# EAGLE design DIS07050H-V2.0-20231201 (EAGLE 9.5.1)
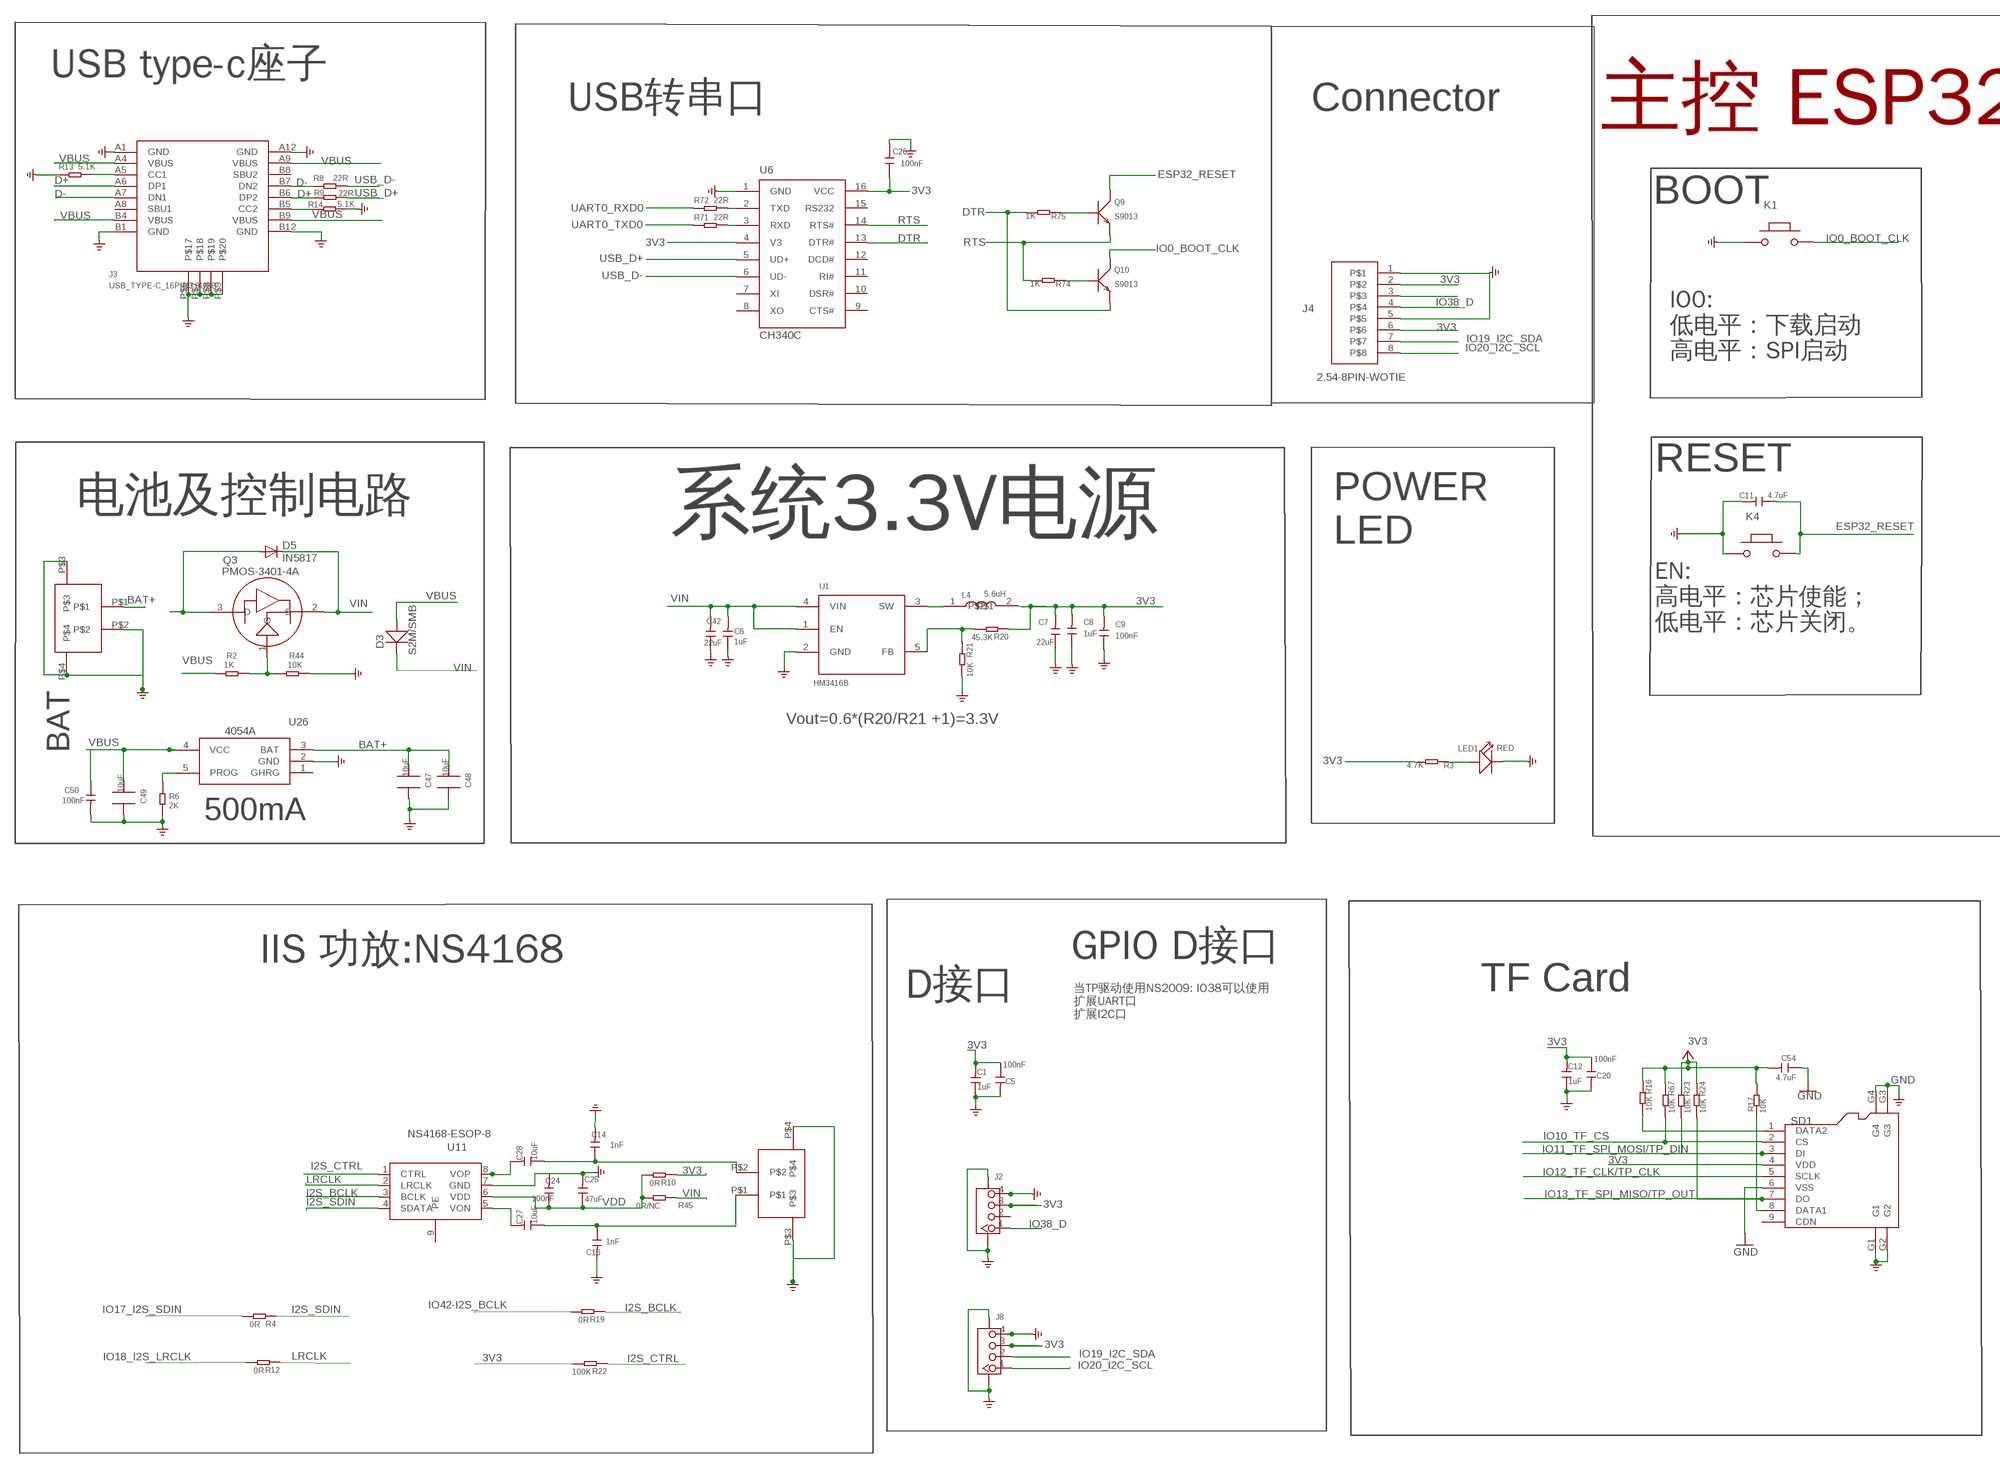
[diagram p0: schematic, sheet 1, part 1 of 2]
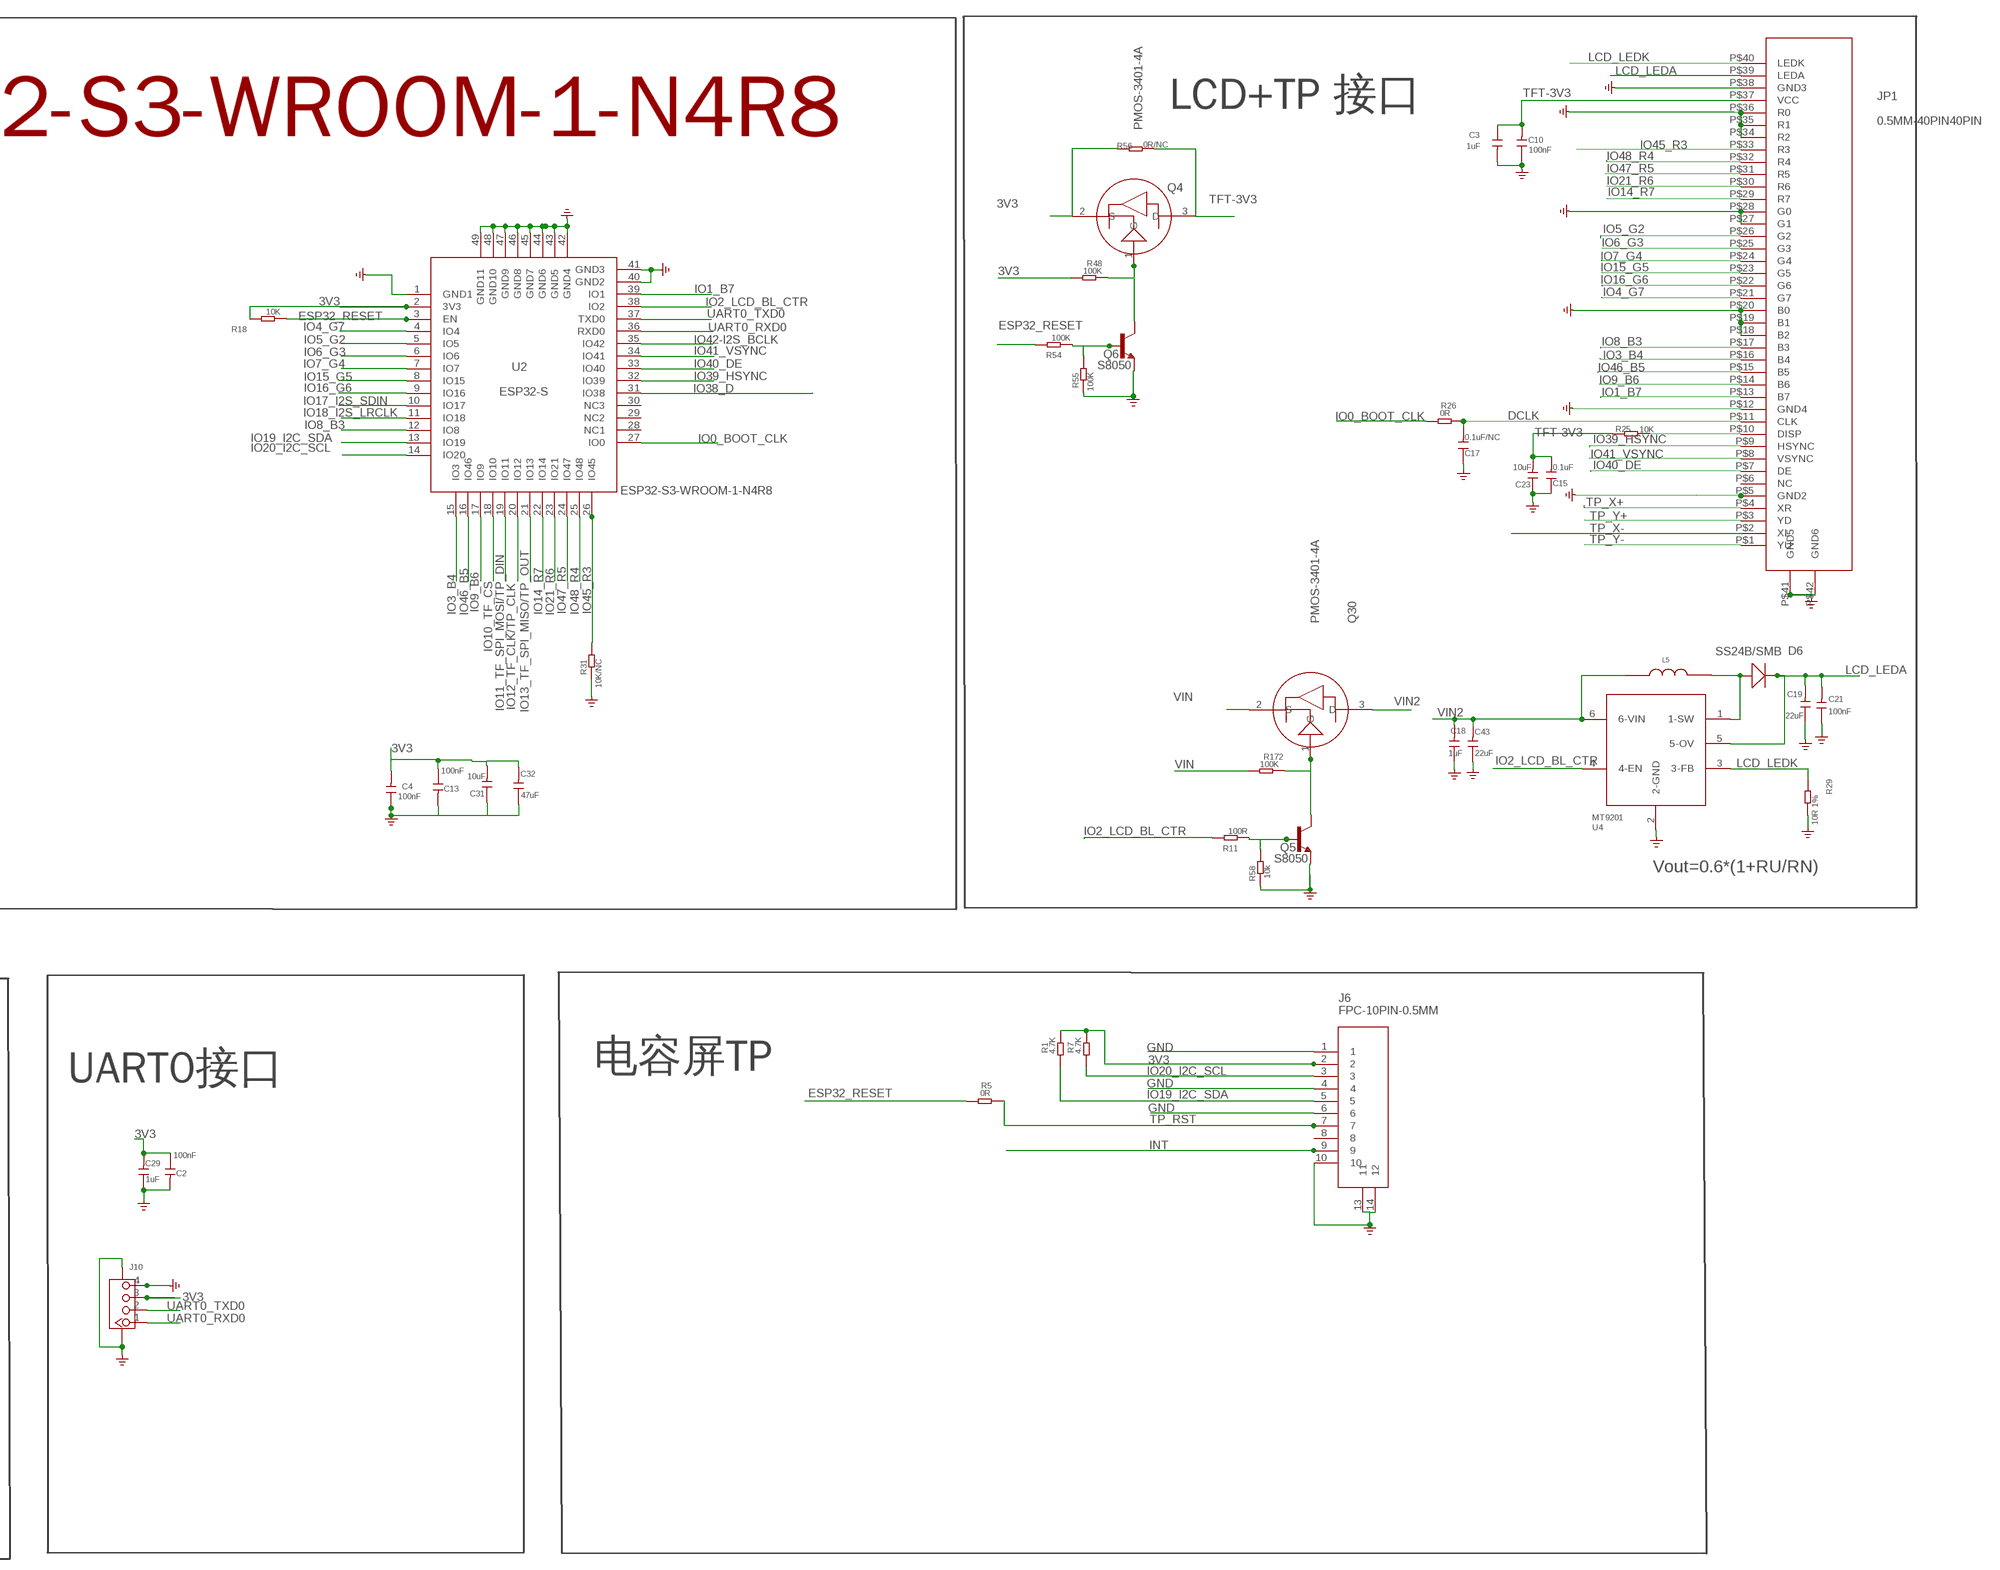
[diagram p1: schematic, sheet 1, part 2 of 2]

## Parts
C1  1uF  DISCRETE_C-0603  [DISCRETE_C0603]
C2  100nF  C-0603  [C0603]
C3  1uF  C-0603  [C0603]
C4  100nF  C-0603  [C0603]
C5  100nF  C-0603  [C0603]
C6  1uF  C0603  [0603]
C7  22uF  C0805  [0805]
C8  1uF  C0603  [0603]
C9  100nF  C0603  [0603]
C10  100nF  C-0603  [C0603]
C11  4.7uF  C0603  [0603]
C12  1uF  DISCRETE_C-0603  [DISCRETE_C0603]
C13  100nF  C-0603  [C0603]
C14  1nF  C-0603  [C0603]
C15  0.1uF  DISCRETE_C-0603  [DISCRETE_C0603]
C16  1nF  C-0603  [C0603]
C17  0.1uF/NC  DISCRETE_C-0603  [DISCRETE_C0603]
C18  1uF  C0603  [0603]
C19  22uF  C0805  [0805]
C20  100nF  C-0603  [C0603]
C21  100nF  C0603  [0603]
C23  10uF  DISCRETE_C-0603  [DISCRETE_C0603]
C24  100nF  C-0603  [C0603]
C25  47uF  C0805  [0805]
C26  100nF  C0603  [0603]
C27  10uF  DISCRETE_C-0603  [DISCRETE_C0603]
C28  10uF  DISCRETE_C-0603  [DISCRETE_C0603]
C29  1uF  DISCRETE_C-0603  [DISCRETE_C0603]
C31  10uF  DISCRETE_C-0603  [DISCRETE_C0603]
C32  47uF  C0805  [0805]
C42  22uF  C0805  [0805]
C43  22uF  C0805  [0805]
C47  10uF  C0805_S  [0805_S]
C48  10uF  C0805_S  [0805_S]
C49  10uF  C0805_S  [0805_S]
C50  100nF  C-0603  [C0603]
C54  4.7uF  DISCRETE_C-0603  [DISCRETE_C0603]
D3  S2M/SMB  214ABDO-214AB  [214AB]
D5  IN5817  DIODE-DO-214AC  [DO-214AC]
D6  SS24B/SMB  214ABDO-214AB  [214AB]
J1  PH2.0WT-2PIN  [PH2.0WT-2PIN]
J2  CONNECTOR_TWIG-4P-2.0-SMD-FEMALE-REINFORCE90D  [CONNECTOR_4P-SMD-2.0-90D]
J3  USB_TYPE-C_16PIN3.0USB  [KEVIN_3.0TYPEC-SMD]
J4  2.54-8PIN-WOTIE  [2.54-8P-WOTIE]
J5  PH2.0WT-2PIN  [PH2.0WT-2PIN]
J6  FPC-10PIN-0.5MM  [FPC-10PIN-0.5MM]
J8  CONNECTOR_TWIG-4P-2.0-SMD-FEMALE-REINFORCE90D  [CONNECTOR_4P-SMD-2.0-90D]
J10  CONNECTOR_TWIG-4P-2.0-SMD-FEMALE-REINFORCE90D  [CONNECTOR_4P-SMD-2.0-90D]
JP1  0.5MM-40PIN40PIN  [0.5MM*40P]
K1  BUTTON  PB157  [157SW]
K4  BUTTON  PB157  [157SW]
L4  5.6uH  L-0530  [CD54_CD54]
L5  CD32_6.8uH  CD32_950MA  [CD32]
LED1  RED  DISCRETE_LED0603  [DISCRETE_LED-0603]
Q3  PMOS-3401-4A  P-MOS-SOT23  [SOT-23]
Q4  PMOS-3401-4A  P-MOS-SOT23  [SOT-23]
Q5  S8050  SPARKFUN_TRANSISTOR_NPNSOT23  [SPARKFUN_SOT23]
Q6  S8050  SPARKFUN_TRANSISTOR_NPNSOT23  [SPARKFUN_SOT23]
Q9  S9013  TRANSISTOR-NPN-SOT23  [SOT23@1]
Q10  S9013  TRANSISTOR-NPN-SOT23  [SOT23@1]
Q30  PMOS-3401-4A  P-MOS-SOT23  [SOT-23]
R1  4.7K  R-0603  [R0603]
R2  1K  DISCRETE_R-0603  [DISCRETE_R0603]
R3  4.7K  DISCRETE_R-0603  [DISCRETE_R0603]
R4  0R  DISCRETE_R-0603  [DISCRETE_R0603]
R5  0R  R-0603  [R0603]
R6  2K  DISCRETE_R-0603  [DISCRETE_R0603]
R7  4.7K  R-0603  [R0603]
R8  22R  DISCRETE_R-0603  [DISCRETE_R0603]
R9  22R  DISCRETE_R-0603  [DISCRETE_R0603]
R10  0R  DISCRETE_R-0603  [DISCRETE_R0603]
R11  100R  R0603  [R0603]
R12  0R  DISCRETE_R-0603  [DISCRETE_R0603]
R13  5.1K  DISCRETE_R-0603  [DISCRETE_R0603]
R14  5.1K  DISCRETE_R-0603  [DISCRETE_R0603]
R16  10K  DISCRETE_R-0603  [DISCRETE_R0603]
R17  10K  DISCRETE_R-0603  [DISCRETE_R0603]
R18  10K  DISCRETE_R-0603  [DISCRETE_R0603]
R19  0R  DISCRETE_R-0603  [DISCRETE_R0603]
R20  45.3K  DISCRETE_R-0603  [DISCRETE_R0603]
R21  10K  DISCRETE_R-0603  [DISCRETE_R0603]
R22  100K  DISCRETE_R-0603  [DISCRETE_R0603]
R23  10K  DISCRETE_R-0603  [DISCRETE_R0603]
R24  10K  DISCRETE_R-0603  [DISCRETE_R0603]
R25  10K  DISCRETE_R-0603  [DISCRETE_R0603]
R26  0R  R-0603  [R0603]
R29  10R 1%  DISCRETE_R-0603  [DISCRETE_R0603]
R31  10K/NC  R0603  [R0603]
R44  10K  DISCRETE_R-0603  [DISCRETE_R0603]
R45  0R/NC  DISCRETE_R-0603  [DISCRETE_R0603]
R48  100K  R-0603  [R0603]
R54  100K  R0603  [R0603]
R55  100K  R0603  [R0603]
R56  0R/NC  DISCRETE_R-0603  [DISCRETE_R0603]
R58  10k  R0603  [R0603]
R67  10K  DISCRETE_R-0603  [DISCRETE_R0603]
R71  22R  DISCRETE_R-0603  [DISCRETE_R0603]
R72  22R  DISCRETE_R-0603  [DISCRETE_R0603]
R74  1K  DISCRETE_R-0603  [DISCRETE_R0603]
R75  1K  DISCRETE_R-0603  [DISCRETE_R0603]
R172  100K  R-0603  [R0603]
SD1  HOLDER-MICROSD-9P  [9P-SMD-W/-RING]
U1  HM3416B  A_XBJ_HM3420B  [A_XBJ_SOT23-5]
U2  ESP32-S  [ESP32-S3]
U4  MT9201  [SOT23-6]
U6  CH340C  CH340G  [SOP-16]
U11  NS4168-ESOP-8  [NS4168-ESOP-8]
U26  4054A  [SOP23-5]

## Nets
3V3: C1.2 C2.1 C4.2 C5.1 C7.2 C8.2 C9.2 C12.2 C13.1 C20.1 C26.1 C29.2 C31.2 C32.2 C54.2 J2.3 J4.2 J4.6 J6.2 J8.3 J10.3 L4.2 Q4.2(S) R1.2 R3.2 R7.2 R10.1 R16.1 R17.1 R18.1 R20.1 R22.2 R23.1 R24.1 R48.1 R56.1 R67.1 SD1.4(VDD) U2.2(3V3) U6.4(V3) U6.16(VCC) ; supply symbol labelled +3V3
BAT+: C47.2 C48.2 D5.A J1.P$1 Q3.3(D) U26.3(BAT)
D+: J3.A6(DP1) J3.B6(DP2) R9.1
D-: J3.A7(DN1) J3.B7(DN2) R8.1
DCLK: C17.2 JP1.P$11(CLK) R26.2
DTR: Q10.2(E) R75.2 U6.13(DTR#)
ESP32_RESET: C11.1 K4.2 Q9.3(C) R5.1 R18.2 R54.2 U2.3(EN)
GND: C1.1 C2.2 C3.2 C4.1 C5.2 C6.1 C7.1 C8.1 C9.1 C10.1 C11.2 C12.1 C13.2 C14.2 C15.1 C16.2 C17.1 C18.1 C19.1 C20.2 C21.1 C23.1 C24.2 C25.2 C26.2 C29.1 C31.1 C32.1 C42.1 C43.1 C47.1 C48.1 C49.1 C50.2 C54.1 J1.P$2 J1.P$3 J1.P$4 J2.4 J2.SS1 J2.SS2 J3.A1(GND) J3.A12(GND) J3.B1(GND) J3.B12(GND) J3.P$6 J3.P$7 J3.P$8 J3.P$9 J4.1 J4.5 J5.P$3 J5.P$4 J6.1 J6.4 J6.6 J6.10 J6.13 J6.14 J8.4 J8.SS1 J8.SS2 J10.4 J10.SS1 J10.SS2 JP1.P$5(GND2) JP1.P$12(GND4) JP1.P$18(B2) JP1.P$19(B1) JP1.P$20(B0) JP1.P$27(G1) JP1.P$28(G0) JP1.P$34(R2) JP1.P$35(R1) JP1.P$36(R0) JP1.P$38(GND3) JP1.P$41(GND5) JP1.P$42(GND6) K1.1 K4.1 LED1.- Q5.2(E) Q6.2(E) R6.2 R13.1 R14.2 R21.2 R29.2 R31.1 R44.1 R55.1 R58.1 SD1.6(VSS) SD1.G1 SD1.G2 SD1.G3 SD1.G4 U1.2(GND) U2.1(GND1) U2.40(GND2) U2.41(GND3) U2.42(GND4) U2.43(GND5) U2.44(GND6) U2.45(GND7) U2.46(GND8) U2.47(GND9) U2.48(GND10) U2.49(GND11) U4.2(2-GND) U6.1(GND) U11.7(GND) U26.2(GND)
I2S_BCLK: R19.1 U11.3(BCLK)
I2S_CTRL: R22.1 U11.1(CTRL)
I2S_SDIN: R4.1 U11.4(SDATA)
INT: J6.9
IO0_BOOT_CLK: K1.2 Q10.3(C) R26.1 U2.27(IO0)
IO1_B7: JP1.P$13(B7) U2.39(IO1)
IO2_LCD_BL_CTR: R11.2 U2.38(IO2) U4.4(4-EN)
IO3_B4: JP1.P$16(B4) U2.15(IO3)
IO4_G7: JP1.P$21(G7) U2.4(IO4)
IO5_G2: JP1.P$26(G2) U2.5(IO5)
IO6_G3: JP1.P$25(G3) U2.6(IO6)
IO7_G4: JP1.P$24(G4) U2.7(IO7)
IO8_B3: JP1.P$17(B3) U2.12(IO8)
IO9_B6: JP1.P$14(B6) U2.17(IO9)
IO10_TF_CS: R67.2 SD1.2(CS) U2.18(IO10)
IO11_TF_SPI_MOSI/TP_DIN: R23.2 SD1.3(DI) U2.19(IO11)
IO12_TF_CLK/TP_CLK: SD1.5(SCLK) U2.20(IO12)
IO13_TF_SPI_MISO/TP_OUT: R24.2 SD1.7(DO) U2.21(IO13)
IO14_R7: JP1.P$29(R7) U2.22(IO14)
IO15_G5: JP1.P$23(G5) U2.8(IO15)
IO16_G6: JP1.P$22(G6) U2.9(IO16)
IO17_I2S_SDIN: R4.2 U2.10(IO17)
IO18_I2S_LRCLK: R12.2 U2.11(IO18)
IO19_I2C_SDA: J4.7 J6.5 J8.2 R1.1 U2.13(IO19)
IO20_I2C_SCL: J4.8 J6.3 J8.1 R7.1 U2.14(IO20)
IO21_R6: JP1.P$30(R6) U2.23(IO21)
IO38_D: J2.1 J4.4 U2.31(IO38)
IO39_HSYNC: JP1.P$9(HSYNC) U2.32(IO39)
IO40_DE: JP1.P$7(DE) U2.33(IO40)
IO41_VSYNC: JP1.P$8(VSYNC) U2.34(IO41)
IO42-I2S_BCLK: R19.2 U2.35(IO42)
IO45_R3: JP1.P$33(R3) R31.2 U2.26(IO45)
IO46_B5: JP1.P$15(B5) U2.16(IO46)
IO47_R5: JP1.P$31(R5) U2.24(IO47)
IO48_R4: JP1.P$32(R4) U2.25(IO48)
LCD_LEDA: C19.2 C21.2 D6.2(-) JP1.P$39(LEDA) U4.5(5-OV)
LCD_LEDK: JP1.P$40(LEDK) R29.1 U4.3(3-FB)
LRCLK: R12.1 U11.2(LRCLK)
N$1: LED1.+ R3.1
N$2: C27.2 U11.5(VON)
N$3: C14.1 C28.1 J5.P$2
N$7: JP1.P$10(DISP) R25.2
N$8: C28.2 U11.8(VOP)
N$11: J3.A5(CC1) R13.2
N$13: L4.1 U1.3(SW)
N$15: C16.1 C27.1 J5.P$1
N$16: D6.1(+) L5.2 U4.1(1-SW)
N$17: J3.B5(CC2) R14.1
N$20: R20.2 R21.1 U1.5(FB)
N$21: Q3.1(G) R2.1 R44.2
N$22: R6.1 U26.5(PROG)
N$23: Q5.1(B) R11.1 R58.2
N$27: Q4.1(G) Q6.3(C) R48.2
N$28: J4.3
N$32: Q9.1(B) R75.1
N$33: Q6.1(B) R54.1 R55.2
N$36: Q5.3(C) Q30.1(G) R172.2
N$38: Q10.1(B) R74.1
N$40: R72.2 U6.2(TXD)
N$42: R71.2 U6.3(RXD)
N$47: R16.2 SD1.1(DATA2)
N$48: R17.2 SD1.8(DATA1)
RTS: Q9.2(E) R74.2 U6.14(RTS#)
TFT-3V3: C3.1 C10.2 C15.2 C23.2 JP1.P$37(VCC) Q4.3(D) R25.1 R56.2
TP_RST: J6.7 R5.2
TP_X+: JP1.P$4(XR)
TP_X-: JP1.P$2(XL)
TP_Y+: JP1.P$3(YD)
TP_Y-: JP1.P$1(YU)
UART0_RXD0: J10.1 R72.1 U2.36(RXD0)
UART0_TXD0: J10.2 R71.1 U2.37(TXD0)
USB_D+: R9.2 U6.5(UD+)
USB_D-: R8.2 U6.6(UD-)
VBUS: C49.2 C50.1 D3.1(+) J3.A4(VBUS) J3.A9(VBUS) J3.B4(VBUS) J3.B9(VBUS) R2.2 U26.4(VCC)
VDD: C24.1 C25.1 R10.2 R45.2 U11.6(VDD)
VIN: C6.2 C42.2 D3.2(-) D5.C Q3.2(S) Q30.2(S) R45.1 R172.1 U1.1(EN) U1.4(VIN)
VIN2: C18.2 C43.2 L5.1 Q30.3(D) U4.6(6-VIN)
Unconnected: J2.2 J3.A8(SBU1) J3.B8(SBU2) J6.8 JP1.P$6(NC) SD1.9(CDN) U2.28(NC1) U2.29(NC2) U2.30(NC3) U6.7(XI) U6.8(XO) U6.9(CTS#) U6.10(DSR#) U6.11(RI#) U6.12(DCD#) U6.15(RS232) U11.9(PE) U26.1(GHRG)

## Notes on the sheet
- USB type-c座子
- USB转串口 | Connector | LCD+TP 接口
- 主控 ESP32-S3-WROOM-1-N4R8
- BOOT
- IO0:
  低电平：下载启动
  高电平：SPI启动
- RESET
- 电池及控制电路
- 系统3.3V电源
- POWER
  LED
- EN:
  高电平：芯片使能；
  低电平：芯片关闭。
- Vout=0.6*(R20/R21 +1)=3.3V
- BAT
- Vout=0.6*(1+RU/RN)
- 500mA
- IIS 功放:NS4168 | GPIO D接口
- TF Card | UART0接口 | 电容屏TP
- D接口
- 当TP驱动使用NS2009: IO38可以使用
  扩展UART口
  扩展I2C口

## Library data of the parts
C1 C12 C27-C29 = A_xbj:DISCRETE_C*: Ceramic Capacitors
C2-C5 C10 C13 C14 C16 C20 C24 C50 = discrete:C*: Ceramic Capacitors
C6 C8 C9 C11 C18 C21 C26 = A_xbj:C0603
C7 C19 C25 C32 C42 C43 = A_xbj:C0805
C15 C17 C23 C31 C54 = A9G:DISCRETE_C*: Ceramic Capacitors
C47-C49 = CPT_SMD:C0805
D3 D6 = DO-214AB:214AB: 214AB
D5 = diode:DIODE-: DIODE
J1 J5 = cooper:PH2.0WT-2PIN
J2 J8 J10 = A_xbj:CONNECTOR_TWIG-4P-2.0-SMD-FEMALE-REINFORCE
J3 = WZ3532R024-ESP32-V0.1-20221226:USB_TYPE-C_16PIN
J4 = cooper:2.54-8PIN-WOTIE
J6 = cooper:FPC-10PIN-0.5MM
JP1 = cooper:0.5MM-40PIN
K1 K4 = MySMD:PB157
L4 = WZ2432R028-ESP32-V1.2-20231108:L-0530
L5 = CD54:CD32_950MA
LED1 = A_xbj:DISCRETE_LED*
Q3 Q4 Q30 = DFN8:P-MOS-SOT23
Q5 Q6 = Adafruit_HUZZAH32_ESP32_Feather:SPARKFUN_TRANSISTOR_NPN: Transistor NPN BJT configuration in SOT23 package. MMBT2222 is the common NPN we use. Double check BCE configuration again layout.
Q9 Q10 = discrete:TRANSISTOR-NPN*: NPN audion
R1 R5 R7 R26 R48 R172 = discrete:R*
R2 R6 R44 = A9G:DISCRETE_R*
R3 R4 R8-R10 R12-R14 R16-R25 R29 R45 R56 R67 R71 R72 R74 R75 = Crowtail-_LED-V2.0-20190615-01:DISCRETE_R*
R11 R31 R54 R55 R58 = cooper:R0603
SD1 = Connector:HOLDER-MICROSD-9P
U1 = CrowBot_-V1.0-20220525:A_XBJ_HM3420B
U2 = DW1000:ESP32-S; U2: ESP32-S3-WROOM-1-N4R8
U4 = cooper:MT9201
U6 = A_xbj:CH340G
U11 = STC_MCUSTC8G1K08A:NS4168-ESOP-8
U26 = DFN8:4054A

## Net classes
0 default: width 0.152 mm, drill 0.305 mm, clearance 0.203 mm

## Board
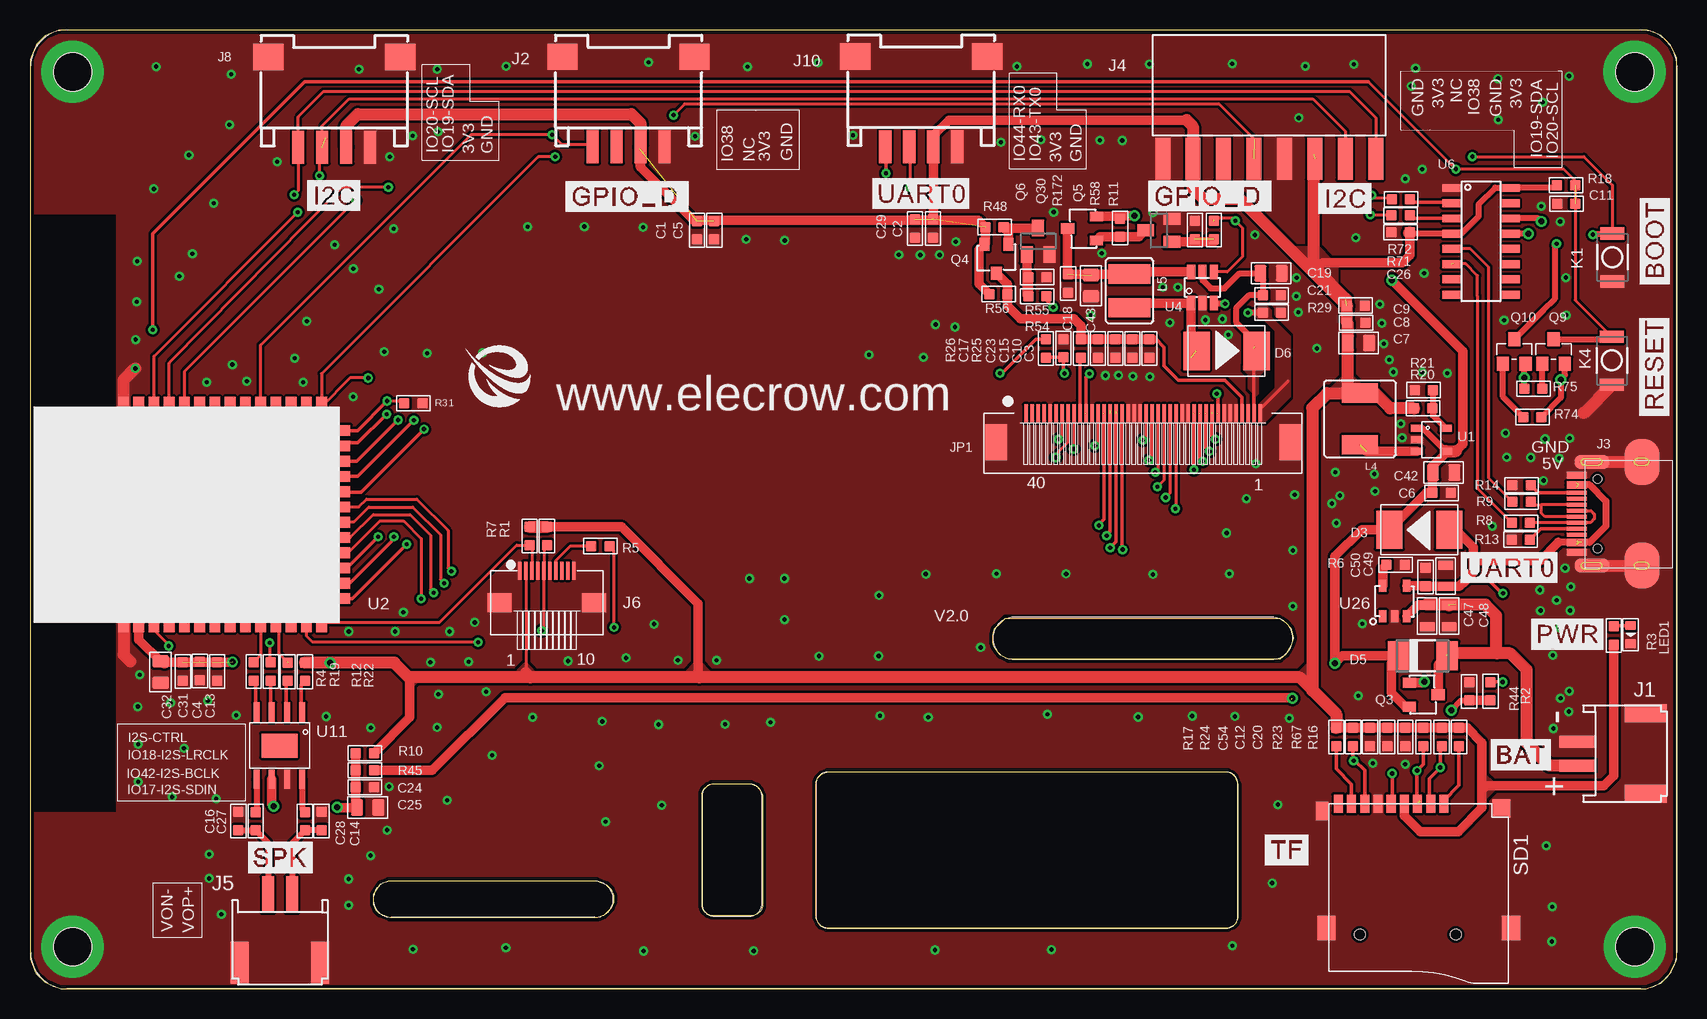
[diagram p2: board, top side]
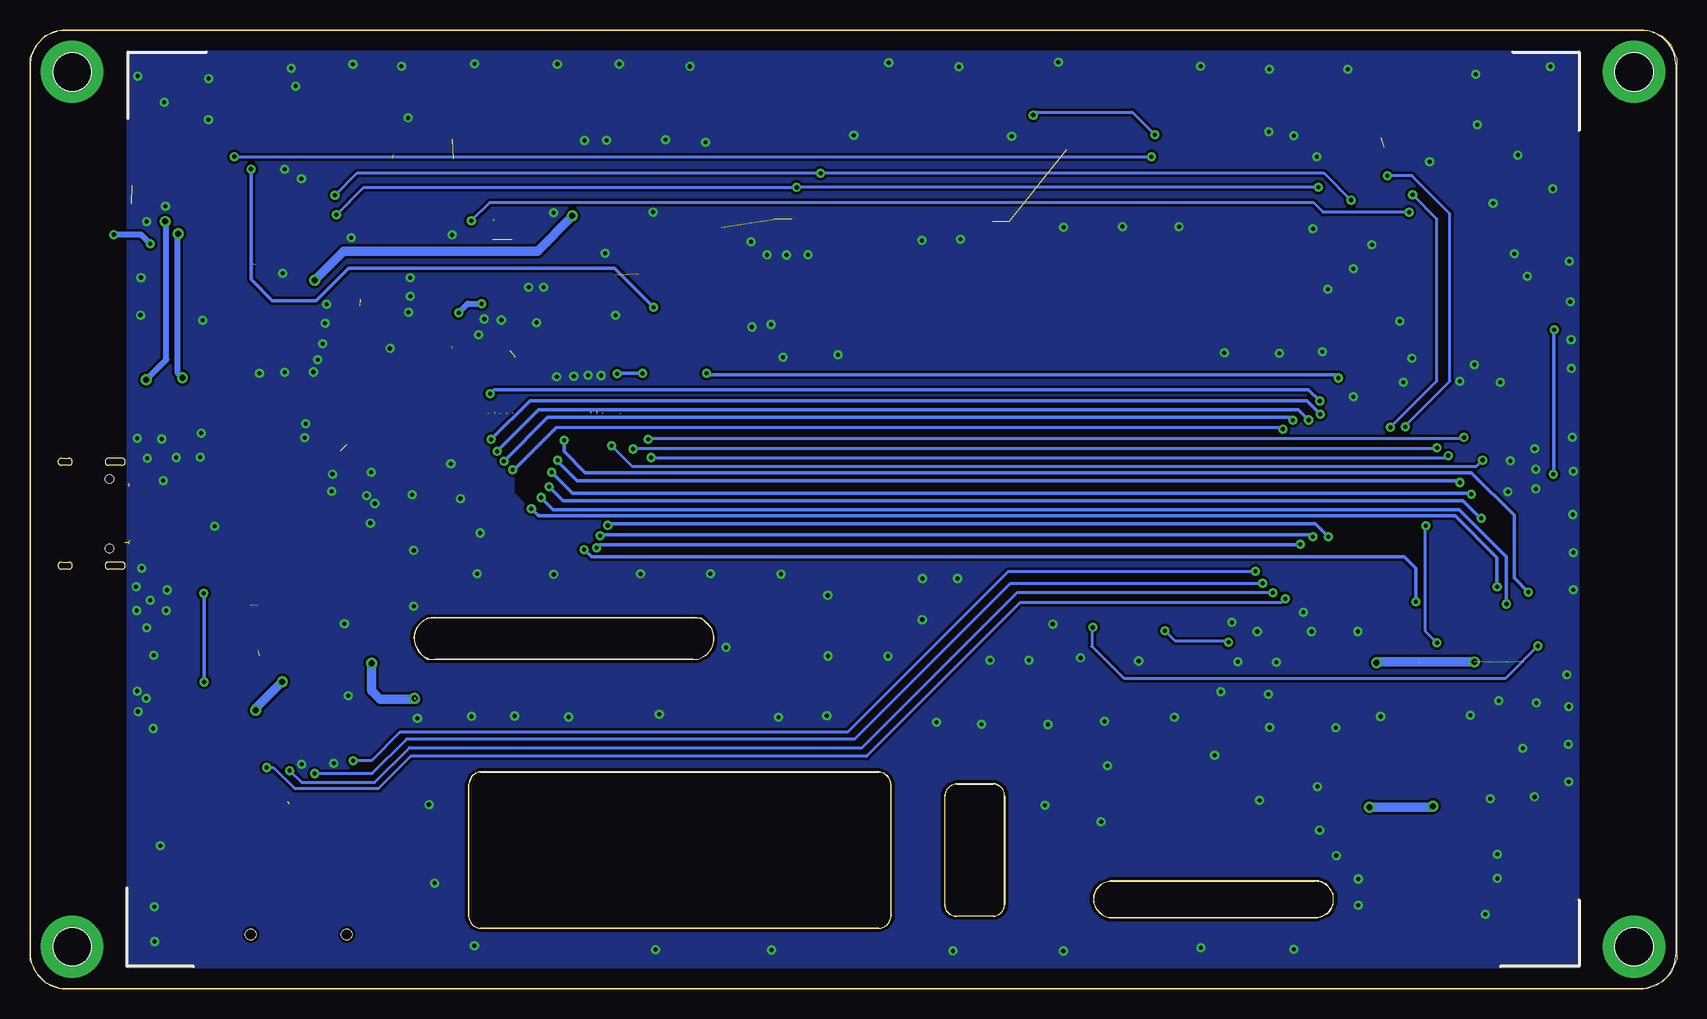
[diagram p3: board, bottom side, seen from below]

Size 137.27 x 79.91 mm. Coordinates in mm from the lower left corner, seen from the top.
Outline: 82 segments
Copper layers (1*16): Top 0.035mm / dielectric 1.5mm / Bottom 0.035mm
Design rules "default *": minimum track width 6mil, minimum drill 0.35mm, track to track 8mil, track to pad 7mil, pad to pad 7mil, via to via 8mil, smd to smd 10mil, copper to edge 10mil, drill to drill 8mil, minimum pad ring 10mil, minimum via ring 8mil, stop-mask expansion 4mil, vias tented up to drill 100mil, thermal gap 0mil

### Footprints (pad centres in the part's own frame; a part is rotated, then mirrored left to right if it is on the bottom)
DISCRETE_C0603 = smd 0.889 x 0.889: 1 -0.762,0; 2 0.762,0
C0603 = smd 0.889 x 0.889: 1 -0.762,0; 2 0.762,0
0603 = smd 0.889 x 0.889: 1 -0.762,0; 2 0.762,0
0805 = smd 1.016 x 1.397: 1 -0.889,0; 2 0.889,0
0805_S = smd 0.762 x 1.27: 1 -0.889,0; 2 0.889,0
214AB = smd 2.2 x 3.2: 1 -2.5,0; 2 2.5,0
DO-214AC = smd 1.8 x 2.4: A 2.025,0; C -2.025,0
PH2.0WT-2PIN = smd 1 x 3: P$1 -1,0; P$2 1,0 | smd 1.5 x 3.5: P$3 -3.35,-5.7; P$4 3.35,-5.7
CONNECTOR_4P-SMD-2.0-90D = smd 1.01 x 2.74: 1 -3,-0.1; 2 -1,-0.1; 3 1,-0.1; 4 3,-0.1 | smd 2.54 x 2.184: SS1 -5.5,7.4; SS2 5.5,7.4
KEVIN_3.0TYPEC-SMD = smd 0.3 x 1.7: A1 -3.35,0.5; A4 -2.55,0.5; A5 -1.25,0.5; A6 -0.25,0.5; A7 0.25,0.5; A8 1.25,0.5; A9 2.55,0.5; A12 3.35,0.5; B1 3.05,0.5; B4 2.25,0.5; B5 1.75,0.5; B6 0.75,0.5; B7 -0.75,0.5; B8 -1.75,0.5; B9 -2.25,0.5; B12 -3.05,0.5 | smd 1.143 x 2.921: P$6 -4.318,-0.762; P$7 4.318,-0.762 | smd 3.81 x 2.921: P$8 -4.318,-4.953; P$9 4.318,-4.953 | hole 0.68: -2.89,-1.22; 2.89,-1.22
2.54-8P-WOTIE = smd 1.25 x 3.5: 1 -8.839,-4.572; 2 -6.35,-4.572; 3 -3.81,-4.572; 4 -1.27,-4.572; 5 1.27,-4.572; 6 3.81,-4.572; 7 6.35,-4.572; 8 8.89,-4.572
FPC-10PIN-0.5MM = smd 0.3 x 1.5: 1 -2.25,2.54; 2 -1.75,2.54; 3 -1.25,2.54; 4 -0.75,2.54; 5 -0.25,2.54; 6 0.25,2.54; 7 0.75,2.54; 8 1.25,2.54; 9 1.75,2.54; 10 2.25,2.54 | smd 2 x 1.6: 13 -3.95,-0.14; 14 3.95,-0.14
0.5MM*40P = smd 0.3 x 1.5: P$1 -8.81,1.73; P$2 -8.31,1.73; P$3 -7.81,1.73; P$4 -7.31,1.73; P$5 -6.81,1.73; P$6 -6.31,1.73; P$7 -5.81,1.73; P$8 -5.31,1.73; P$9 -4.81,1.73; P$10 -4.31,1.73; P$11 -3.81,1.73; P$12 -3.31,1.73; P$13 -2.81,1.73; P$14 -2.31,1.73; P$15 -1.81,1.73; P$16 -1.31,1.73; P$17 -0.81,1.73; P$18 -0.31,1.73; P$19 0.19,1.73; P$20 0.69,1.73; P$21 1.19,1.73; P$22 1.69,1.73; P$23 2.19,1.73; P$24 2.69,1.73; P$25 3.19,1.73; P$26 3.69,1.73; P$27 4.19,1.73; P$28 4.69,1.73; P$29 5.19,1.73; P$30 5.69,1.73; P$31 6.19,1.73; P$32 6.69,1.73; P$33 7.19,1.73; P$34 7.69,1.73; P$35 8.19,1.73; P$36 8.69,1.73; P$37 9.19,1.73; P$38 9.69,1.73; P$39 10.19,1.73; P$40 10.69,1.73 | smd 1.8 x 3: P$41 -11.31,-0.67; P$42 13.19,-0.67
157SW = smd 1.016 x 1.981: 1 0,0; 2 4,0
CD54_CD54 = smd 3 x 1.6: 1 0,2.159; 2 0,-2.159
CD32 = smd 3.5 x 1.6: 1 0,1.409; 2 0,-1.409
DISCRETE_LED-0603 = smd 0.762 x 0.889: + -0.762,0; - 0.762,0
SOT-23 = smd 1.1 x 0.8: 1 1.2,-1; 2 1.2,1 | smd 1.1 x 0.9: 3 -1.2,0
SPARKFUN_SOT23 = smd 1 x 1.4: 1 -0.95,-1.1; 2 0.95,-1.1; 3 0,1.1
SOT23@1 = smd 1.016 x 1.143: 1 -0.95,-1.016; 2 0.95,-1.016; 3 0,1.016
R0603 = smd 0.889 x 0.889: 1 -0.762,0; 2 0.762,0
DISCRETE_R0603 = smd 0.889 x 0.889: 1 -0.762,0; 2 0.762,0
9P-SMD-W/-RING = smd 1.524 x 0.762: 1 0,4.4; 2 0,3.3; 3 0,2.2; 4 0,1.1; 5 0,0; 6 0,-1.1; 7 0,-2.2; 8 0,-3.3; 9 0,-4.4 | smd 1.524 x 1.016: G1 0.6,-5.746 | smd 2.032 x 1.524: G2 10.373,-5.4; G3 10.373,10 | smd 1.524 x 1.524: G4 0.392,9.181 | hole 0.889: 10.9,-2.6; 10.9,5.4
A_XBJ_SOT23-5 = smd 0.6 x 1: 1 -0.95,-1.2; 2 0,-1.2; 3 0.95,-1.2; 4 0.95,1.2; 5 -0.95,1.2
ESP32-S3 = smd 1.6 x 0.9: 1 0,18.01; 2 0,16.74; 3 0,15.47; 4 0,14.2; 5 0,12.93; 6 0,11.66; 7 0,10.39; 8 0,9.12; 9 0,7.85; 10 0,6.58; 11 0,5.31; 12 0,4.04; 13 0,2.77; 14 0,1.5; 27 18,1.5; 28 18,2.77; 29 18,4.04; 30 18,5.31; 31 18,6.58; 32 18,7.85; 33 18,9.12; 34 18,10.39; 35 18,11.66; 36 18,12.93; 37 18,14.2; 38 18,15.47; 39 18,16.74; 40 18,18.01 | smd 0.9 x 1.8: 15 2,0; 16 3.28,0; 17 4.55,0; 18 5.82,0; 19 7.09,0; 20 8.36,0; 21 9.63,0; 22 10.9,0; 23 12.17,0; 24 13.44,0; 25 14.71,0; 26 16,0 | smd 1 x 1: 41 7.64,11.16; 42 9.14,11.16; 43 6.14,11.16; 44 6.14,14.16; 45 7.64,12.66; 46 9.14,12.66; 47 7.64,14.16; 48 9.14,14.16; 49 6.14,12.66
SOT23-6 = smd 0.69 x 1.2: 1 -0.95,-1.3; 2 0,-1.3; 3 0.95,-1.3; 4 0.95,1.3; 5 0,1.3; 6 -0.95,1.3
SOP-16 = smd 0.66 x 1.5: 1 -4.445,-2.475; 2 -3.175,-2.475; 3 -1.905,-2.475; 4 -0.635,-2.475; 5 0.635,-2.475; 6 1.905,-2.475; 7 3.175,-2.475; 8 4.445,-2.475; 9 4.445,2.475; 10 3.175,2.475; 11 1.905,2.475; 12 0.635,2.475; 13 -0.635,2.475; 14 -1.905,2.475; 15 -3.175,2.475; 16 -4.445,2.475
NS4168-ESOP-8 = smd 1.6 x 0.5: 1 -2.8,1.905; 2 -2.8,0.635; 3 -2.8,-0.635; 4 -2.8,-1.905; 5 2.8,-1.905; 6 2.8,-0.635; 7 2.8,0.635; 8 2.8,1.905 | smd 2 x 3: 9 0,0
SOP23-5 = smd 1 x 0.635: 1 -1.27,1; 2 -1.27,0; 3 -1.27,-1; 4 1.27,-1; 5 1.27,1

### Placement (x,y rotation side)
C1  55.61,63.22 90 top
C2  75.26,63.36 270 top
C3  93.32,53.37 270 top
C4  14.17,26.48 90 top
C5  57.04,63.22 270 top
C6  117.67,41.33 180 top
C7  110.74,53.82 180 top
C8  110.54,55.51 180 top
C9  110.52,56.94 180 top
C10  91.9,53.37 90 top
C11  128.07,65.42 180 top
C12  113.15,20.99 90 top
C13  15.61,26.44 270 top
C14  24.29,13.99 90 top
C15  90.47,53.37 90 top
C16  17.37,13.99 90 top
C17  86.15,53.4 270 top
C18  86.54,58.78 90 top
C19  103.45,59.63 180 top
C20  114.65,20.99 270 top
C21  103.52,57.79 180 top
C23  89.03,53.37 90 top
C24  27.91,16.8 0 top
C25  28.15,15.11 0 top
C26  114.26,63.05 180 top
C27  18.81,13.97 90 top
C28  22.92,13.97 90 top
C29  73.76,63.36 90 top
C31  12.74,26.45 90 top
C32  10.89,26.4 90 top
C42  117.84,43.03 180 top
C43  88.44,58.6 90 top
C47  116.46,31.08 90 top
C48  118.29,31.07 90 top
C49  118.01,34.42 270 top
C50  116.33,34.32 90 top
C54  111.71,20.99 90 top
D3  115.81,38.26 180 top
D5  116.1,27.75 0 top
D6  99.74,53.16 0 top
J1  128.97,19.61 90 top
J2  49.9,70.28 0 top
J3  129.44,39.6 90 top
J4  103.29,73.77 0 top
J5  20.83,7.88 0 top
J6  43.08,32.31 0 top
J8  25.36,70.25 0 top
J10  74.29,70.29 0 top
JP1  91.84,46.23 0 top
K1  131.9,58.95 90 top
K4  131.86,50.34 90 top
L4  110.87,47.5 180 top
L5  91.67,58.17 0 top
LED1  133.43,29.52 270 top
Q3  116.18,24.51 180 top
Q4  80.56,60.85 90 top
Q5  94.1,63.22 90 top
Q6  84.04,62.3 0 top
Q9  127,53.12 0 top
Q10  123.72,53.12 0 top
Q30  87.7,63.37 0 top
R1  43.08,37.74 90 top
R2  121.74,24.8 90 top
R3  132.03,29.46 270 top
R4  18.66,26.45 90 top
R5  47.54,36.9 180 top
R6  113.84,35.36 0 top
R7  41.66,37.74 90 top
R8  124.27,38.85 180 top
R9  124.32,40.59 180 top
R10  27.91,19.64 180 top
R11  98.69,63.24 90 top
R12  21.47,26.43 90 top
R13  124.27,37.45 0 top
R14  124.33,41.98 180 top
R16  119.12,20.99 270 top
R17  108.89,20.99 270 top
R18  128.05,66.96 0 top
R19  20.08,26.45 90 top
R20  116.12,48.38 0 top
R21  116.18,49.9 180 top
R22  22.92,26.43 90 top
R23  116.15,20.99 270 top
R24  110.28,20.99 270 top
R25  87.6,53.37 270 top
R26  84.68,53.37 270 top
R29  103.52,56.36 0 top
R31  31.97,48.8 180 top
R44  119.96,24.8 270 top
R45  27.91,18.22 180 top
R48  80.4,63.48 0 top
R54  83.97,57.72 0 top
R55  83.98,59.32 180 top
R56  80.73,57.91 0 top
R58  97.09,63.24 270 top
R67  117.68,20.99 270 top
R71  114.25,64.45 0 top
R72  114.28,65.8 0 top
R74  125.24,47.66 0 top
R75  125.32,50.01 180 top
R172  90.87,63.42 270 top
SD1  113.46,15.44 270 top
U1  116.81,45.76 270 top
U2  25.81,30.53 90 top
U4  97.74,58.45 0 top
U6  120.95,62.3 270 top
U11  20.8,20.27 270 top
U26  113.76,32.32 90 top
U$30  [ELECROW-NEW]  36.28,48.48 0 top
U$33  [5.0底框]  138.34,-0.06 0 bottom
U$41  [5.0板框]  -0.6,0.03 0 top

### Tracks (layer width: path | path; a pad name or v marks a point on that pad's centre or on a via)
0
  cutout Bottom: 93.15,46.48 96.51,46.48 96.76,46.23 96.76,41.36 95.08,39.68 95.08,41.78 93.06,43.79 93.06,46.4
3V3  (via drill 0.5)  (9 unrouted)
  Top 0.203: 109.65,56.95 C9.2 109.53,56.83 | C8.2 109.55,55.54
  Top 0.254: J6.2 41.33,26.31 41.33,25.97 41.4,25.9
  Top 0.5: U6.16 123.45,66.77 | C26.1 115.13,62.93 U6.4 119.32,62.93 120.75,64.36 120.75,65.37 122.15,66.77 123.45,66.77 | R18.1 127.09,66.77 123.45,66.77
  Top 0.8: C32.2 9.07,29.12 U2.2 | SD1.4 114.56,14.45 115.9,13.11 119.04,13.11 121.04,15.1 121.04,16.58 | 50.85,69.96 50.85,68.53 50.9,68.48 | J10.3 75.32,70.23 | 75.32,70.23 75.32,64.18 C2.1 | 96.42,72.4 76.6,72.4 75.32,71.12 75.32,70.23 | 50.9,68.48 55.32,64.06 79.06,64.06 R48.1 79.64,62.13 Q4.2 79.1,61.59 79.1,58.77 R56.1 | 50.9,68.48 J2.3 | R17.1 R24.1 C54.2 C12.2 C20.1 R23.1 R67.1 R16.1 119.81,21.75 121.04,20.52 121.04,16.58 | R1.2 43.67,38.51 43.68,38.5 49.3,38.5 55.68,32.12 55.68,26.07 55.8,25.95 55.85,25.9 | v16.88,27.24 16.84,27.21 11.23,27.21 | 31.66,25.9 31.66,22.63 R10.1 | 121.04,16.58 121.4,16.94 131.19,16.94 132.03,17.78 R3.2 | 107.22,59.96 107.77,60.51 114.4,60.51 115.02,61.13 C26.1
  Top 1: 11.23,27.21 11.14,27.29 C32.2 | 114.97,63 C26.1 | R22.2 v25.02,27.19 30.37,27.19 31.66,25.9 31.71,25.95 41.7,25.95 | R7.2 R1.2 | 109.71,57.47 107.22,59.96 107.01,60.17 107.01,69.52 | 110.37,49.66 109.85,50.18 C7.2 109.85,55.44 C8.2 109.78,56.92 C9.2 100.91,65.79 97.87,65.79 96.94,66.72 J4.2 96.94,71.88 96.42,72.4 | J8.3 26.36,71.93 27.33,72.9 50.14,72.9 50.9,72.14 J2.3 | 41.7,25.95 55.8,25.95 105.85,25.95 108.89,22.91 R17.1 108.89,22.87 106.88,24.87 106.88,48.41 108.13,49.66 110.37,49.66 | 41.7,25.95 41.33,26.31 | 110.37,49.66 L4.2 | R20.1 113.39,48.38 112.07,49.71 110.42,49.71 110.37,49.66
  Bottom 0.8: v25.02,27.19 24.97,27.24 v16.88,27.24 | v16.88,27.24
  pour Top (no thermals): 107.09,60.26 109.02,60.26 109.02,58.24 107.09,60.17
  pour Top (no thermals): 106.67,27.33 105.41,26.07 106.84,24.64 106.84,27.41 106.76,27.41
  pour Top (no thermals): 31.49,24.72 32.42,25.65 31.49,26.57
  pour Top (no thermals): 121.12,15.57 122.38,16.83 120.95,18.26 120.95,15.48 121.04,15.48
  pour Top (no thermals): 56.94,26.24 55.68,27.5 54.26,26.07 57.03,26.07 57.03,26.15
  pour Top (no thermals): 42.58,25.98 41.32,27.24 39.89,25.82 42.66,25.82 42.66,25.9
  pour Top (no thermals): 111.12,50.26 109.86,51.52 108.44,50.09 111.21,50.09 111.21,50.18
  pour Top (no thermals): 105.09,61.91 107.02,61.91 107.02,59.89 105.09,61.82
  pour Top (no thermals): 108.91,60.32 106.98,60.32 106.98,62.33 108.91,60.4
BAT+  (2 unrouted)
  Top 0.8: C48.2 118.3,31.96 | C47.2 115.68,31.97 U26.3 115.72,32.01 116.43,32.01 | 118.87,32.01 118.29,32.01 | Q3.3 117.38,27.01 D5.A
  Top 1: J1.P$1 126.65,18.61 124.75,20.5 124.75,26.6 123.39,27.97 122.3,27.97 | 122.3,27.97 118.26,27.97 118.26,28.17 | 122.3,27.97 122.23,28.04 122.23,31.11 121.33,32.01 118.29,32.01 | C48.2 118.24,32.01 116.43,32.01
D+
  Top 0.254: J3.A6 126.29,39.35 125.98,39.65 125.98,40.3 | J3.B6 125.98,40.34 125.98,40.3 | 125.98,40.3 125.37,40.3 R9.1
D-
  Top 0.254: R8.1 J3.B7 130.09,38.85 130.4,39.17 130.4,39.57 130.13,39.85 J3.A7
DCLK  (via drill 0.35)  (1 unrouted)
  Top 0.3: R26.2 84.71,52.63 C17.2 86.16,51.35 v86.22,51.29 | v88.32,51.26 88.03,50.97 88.03,47.91
  Bottom 0.3: v88.32,51.26 88.3,51.29 v86.22,51.29
DTR  (via drill 0.5)
  Top 0.5: R75.2 v124.56,50.93 124.56,51.98 Q10.2 | v124.9,62.94 124.89,62.93 U6.13
  Bottom 0.5: v124.9,62.94 124.98,62.87 124.98,51.35 v124.56,50.93
ESP32_RESET  (via drill 0.35)  (1 unrouted)
  Top 0.152: 131.84,54.36 K4.2
  Top 0.254: K4.2 128.81,57.39 R18.2 128.81,67.35 127.84,68.32 v118.85,68.32 111.56,75.61 | U2.3 10.34,29.9 11.57,28.66 v11.57,28.58 | R5.1 48.63,36.57 48.63,30.17 v48.68,30.12
  Top 0.3: v10.28,42.89 10.28,30.59 U2.3 | 111.56,75.61 22.88,75.61 10.22,62.95 v10.22,54.92 | v85.29,56.81 84.74,57.37 R54.2
  Top 0.5: Q9.3 131.65,54.13 K4.2
  Bottom 0.254: v48.68,30.12 48.76,30.2 48.76,28.55 46.1,25.89 14.26,25.89 v11.57,28.58
  Bottom 0.3: v10.28,42.89 10.26,42.91 10.26,54.88 v10.22,54.92 | v118.85,68.32 118.85,59.13 117.07,57.35 113.41,57.35 110.72,60.05 88.53,60.05 v85.29,56.81
GND  (via drill 0.35, 3.2 pad 5.2)
  Top 1: v8.78,51.7 7.8,50.72 U2.40 7.8,45.62 8.1,45.31 | 7.9,33.3 7.8,33.2 U2.1 7.8,27.87 8.38,27.28 | J3.P$7 J3.P$9 | J3.P$6 J3.P$8 | K4.1 129.51,47.99
  other vias: 133.76,76.43 3.56,76.43 3.56,3.51 133.77,3.51 91.94,51.05 75.83,61.17 127.55,63.94 105.27,36.54 52.66,15.32 115.13,75.23 22.78,50.56 69.93,52.84 100.23,3.6 102.09,62.83 82.26,76.87 13.54,61.26 95.03,55.53 84.81,22.88 55.44,71.06 126.16,42.36 29.99,69.34 11.86,16 106.31,76.89 46.21,63.53 41.89,22.63 65.76,27.74 99.75,37.99 15.96,6.21 9.02,17.25 105.28,31.9 26.95,49.35 26.55,9.16 89.19,70.73 126.29,45.83 105.56,57.73 85.13,3.28 100.22,77.11 113.64,51.41 89.66,51.11 14.83,24.02 127.49,44.22 74.87,22.63 91.05,70.7 88.14,77.08 114.28,47.1 111.06,30.42 92.38,22.66 27.42,76.63 115.5,76.73 93.36,51.02 74.49,52.64 34.01,71.43 30.32,63.34 75.45,3.24 93.31,77.07 33.11,52.96 108.52,40.45 47.7,22.29 33.95,76.64 88.45,56.13 123.09,44.3 77.17,62.27 29.08,58.31 57.95,22.06 110.73,24.44 122.39,72.44 93.61,34.54 65.69,77.18 100.45,22.71 13.86,44 39.69,76.88 33.38,27.23 72.42,61.19 112.12,41.46 105.72,56.39 8.99,23.53 90.75,51.14 102.19,43.77 29.54,53.1 126.99,21.7 8.81,54.11 52.01,30.41 52.41,22.04 74.21,61.16 128.38,31.53 116.05,68.32 128.34,45.89 15.31,65.47 24.68,22.7 47.45,18.59 101.39,40.86 38.52,19.47 99.99,34.61 70.75,27.74 34.05,24.55 70.85,22.76 13.25,69.49 11.72,23.83 26.56,6.98 17.2,22.79 125.98,65.22 33.93,21.79 20.61,68.93 41.48,63.52 38.01,24.77 59.82,76.85 28.41,21.77 80.56,34.59 79.25,28.46 59.7,62.46 112.05,42.9 114.38,45.92 8.63,33.26 8.63,36.36 8.68,39.53 8.63,43.14 8.7,45.96 95.69,58.46 97.97,55.74 99.4,55.82 77.09,55.16 75.5,55.37 51.55,77.23 109.2,41.11 99.88,54.5 94.45,58.46 14.07,41.42 47.98,13.92 11.75,43.32 49.69,27.58 11.74,41.66 9.03,20.4 12.84,20.06 8.89,57.27 128.26,23.11 8.95,60.64 128.32,24.82 12.46,59.38 59.97,34.2 9.15,26.17 108.82,43.06 31.12,31.4 112.87,53.77 15.53,15.84 54,27.39 62.91,62.37 108.89,38.82 14.95,11.22 126.95,27.8 14.94,9.21 104.01,15.36 39.66,3.43 51.14,3.16 31.92,3.32 70.77,32.79 111.94,18.81 74.67,34.57 85.33,64.74 61.72,22.22 16.63,72 62.9,30.78 80.95,70.56 31.9,71.11 107.26,53.37 114.64,67.51 93.62,64.68 105.58,59.27 84.28,70.75 125.09,44.28 16.77,76.23 126.09,73.88 122.99,46.32 128.02,59.28 128.05,56.15 122.88,55.72 37.72,53.02 68.6,71.14 36.57,27.27 60.33,3.17 51.11,63.48 86.37,34.58 28.39,11.11 44.85,27.32 62.88,34.2 121.88,38.55 126.86,3.95 127.58,24.23 103.55,8.82 122.37,75.86 110.35,77.06 116.21,59.65 112.53,57.04 112.68,55.47 10.53,76.86 10.33,66.66 127.53,30.09 105.42,41.18 128.43,33.52 125.85,33.24 127.25,32.39 125.91,31.53 127.96,35.07 126.4,11.92 126.9,6.85 26.96,60.02 22.07,52.56 23.08,55.63 89.34,61.3 128.3,76.07 34.77,15.73 37.08,30.54 30.44,29.79 34.98,29.79 26.58,29.79 29.77,13.24 29.95,16.86 11.85,45.01 114.63,18.73 104.98,22.56 96.88,22.74 118.15,51.3 113.3,52.43 116.05,51.39 14.72,50.56 18.08,50.64 16.87,52.03 25.4,62.01 110.51,62.6 105.76,72.58 57.23,27.38
  pour Bottom: 8.19,78.05 129.11,78.05 129.11,1.84 8.19,1.84
  pour Top (rank 4): -0.01,79.91 137.25,79.91 137.25,-0.06 -0.09,-0.06 -0.09,14.73 7.22,14.73 7.22,64.54 -0.01,64.54
I2S_BCLK
  Top 0.3: U11.3 20.08,23.15 R19.1
I2S_CTRL
  Top 0.3: U11.1 22.62,23.15 22.62,25.36 R22.1
I2S_SDIN
  Top 0.3: U11.4 18.81,23.15 18.81,25.54 R4.1
IO0_BOOT_CLK  (via drill 0.35)
  Top 0.254: v43.79,69.33 42.36,69.33 24.31,51.28 U2.27 26.69,50.91 v28.2,50.91 | v120.23,69.36 129.53,69.36 131.9,66.99 K1.2
  Top 0.3: v80.87,51.3 81.03,51.3 83.87,54.13 R26.1
  Top 0.5: Q10.3 126.16,56.57 127.08,57.49 127.08,61.94 v127.25,62.1 | v130.28,62.86 130.36,62.94 132.29,62.94 132.28,62.95 K1.2
  Bottom 0.254: v120.23,69.36 v120.23,69.35 43.81,69.35 v43.79,69.33
  Bottom 0.3: v80.87,51.3 80.73,51.16 28.45,51.16 v28.2,50.91
  Bottom 0.5: v127.25,62.1 128.01,62.86 v130.28,62.86
IO1_B7  (via drill 0.35)
  Top 0.254: JP1.P$13 89.03,45.34 88.94,45.25 v88.79,45.25 | U2.39 9.07,47.14 10.16,46.05 14.2,46.05 v16.19,44.07
  Bottom 0.254: v88.79,45.25 87.1,43.56 16.69,43.56 v16.19,44.07 | v16.19,44.07
IO2_LCD_BL_CTR  (via drill 0.35)  (1 unrouted)
  Top 0.254: v22.31,64.72 10.34,52.74 U2.38 | 98.59,64.11 98.69,64.21 100.28,64.21 v100.48,64 101.07,63.41 101.08,63.41 101.08,61.03 99.81,59.75 U4.4
  Bottom 0.254: v22.31,64.72 29.47,64.72 30.3,65.55 98.94,65.55 v100.48,64
IO3_B4  (via drill 0.35)  (1 unrouted)
  Top 0.3: 90.52,48.14 90.52,37.24 v90.04,36.76 | U2.15 26.85,32.53 v31.39,37.07
  Bottom 0.3: v90.04,36.76 89.79,37.01 31.44,37.01 v31.39,37.07
IO4_G7  (via drill 0.35)
  Top 0.254: v92.76,45.72 93.03,45.99 JP1.P$21
  Top 0.3: U2.4 11.61,32.31 v12.37,33.07
  Bottom 0.3: v12.37,33.07 13.55,34.25 13.55,39.45 17.12,43.03 91,43.03 92.76,44.79 v92.76,45.72
IO5_G2  (via drill 0.35)
  Top 0.254: JP1.P$26 95.53,40.05 v95.48,40
  Top 0.3: U2.5 12.88,32.25 14.14,33.51 v14.98,33.51
  Bottom 0.3: v14.98,33.51 14.98,35.94 18.45,39.42 94.89,39.42 v95.48,40
IO6_G3  (via drill 0.35)
  Top 0.254: JP1.P$25 95.03,41.31 v94.67,40.95
  Top 0.3: U2.6 14.15,32.03 v14.19,32.07
  Bottom 0.3: v14.19,32.07 14.19,36.02 18.11,39.94 93.66,39.94 v94.67,40.95
IO7_G4  (via drill 0.35)
  Top 0.254: JP1.P$24 94.53,42.4 v93.99,41.86
  Top 0.3: v16.29,39.22 16.29,33.59 15.42,32.72 U2.7
  Bottom 0.3: v93.99,41.86 92.81,40.68 17.84,40.68 16.38,39.22 v16.29,39.22
IO8_B3  (via drill 0.35)
  Top 0.3: v21.74,32.27 21.77,32.25 U2.12 | JP1.P$17 91.03,36.61 v91.08,36.61
  Bottom 0.3: v91.08,36.61 90.48,36 22.7,36 21.74,35.05 v21.74,32.27
IO9_B6  (via drill 0.35)  (1 unrouted)
  Top 0.3: U2.17 26.44,35.08 v29.03,37.67 | v89.1,38.62 89.1,38.71 89.52,39.12 89.52,47.94
  Bottom 0.3: v89.1,38.62 88.96,38.76 30.12,38.76 v29.03,37.67
IO10_TF_CS  (via drill 0.35)
  Top 0.254: U2.18 26.54,36.35 29.18,39 31.13,39 32.61,37.52 v32.61,32.51
  Top 0.3: SD1.2 116.63,15.56 116.63,17.53 v117.55,18.45 117.55,20.1 R67.2
  Bottom 0.254: v117.55,18.45 116.96,18.45 115.21,16.7 108.2,16.7 105.52,19.38 67.54,19.38 54.71,32.21 32.92,32.21 v32.61,32.51
IO11_TF_SPI_MOSI/TP_DIN  (via drill 0.35)  (1 unrouted)
  Top 0.254: U2.19 26.7,37.62 28.61,39.53 31.67,39.53 33.38,37.82 33.38,33.3 v33.66,33.02
  Top 0.3: R23.2 116.15,18.73 v115.62,18.19 115.62,15.88 115.85,15.65
  Bottom 0.254: v115.62,18.19 114.63,17.2 108.53,17.2 105.63,20.1 67.91,20.1 54.99,33.02 v33.66,33.02
IO12_TF_CLK/TP_CLK  (via drill 0.35)
  Top 0.254: U2.20 26.98,38.89 28.24,40.15 31.91,40.15 34.21,37.85 34.21,34.11 v34.52,33.81
  Top 0.3: SD1.5 113.54,15.52 v113.54,17.95
  Bottom 0.254: v113.54,17.95 108.75,17.95 105.89,20.81 68.54,20.81 55.55,33.8 v34.52,33.8 v34.52,33.81
IO13_TF_SPI_MISO/TP_OUT  (via drill 0.35)
  Top 0.254: U2.21 27.4,40.16 28.06,40.82 32.23,40.82 34.85,38.2 34.85,35.08 v35.13,34.8
  Top 0.3: R24.2 110.28,19.02 v110.33,19.02 110.44,19.02 111.26,18.21 SD1.7
  Bottom 0.254: v110.33,19.02 108.81,19.02 106.45,21.39 69.14,21.39 55.73,34.8 v35.13,34.8
IO14_R7  (via drill 0.35)  (1 unrouted)
  Top 0.3: U2.22 25.89,41.35 26.14,41.35 26.2,41.4 27.59,41.4 v32.84,46.65 | 97.01,47.96 97.01,43.27 v97.03,43.26
  Bottom 0.254: 93.45,46.73 93.4,46.78 32.98,46.78 v32.84,46.65
  Bottom 0.3: v97.03,43.26 96.93,43.26 93.45,46.73 | v32.84,46.65 32.93,46.73
IO15_G5  (via drill 0.35)
  Top 0.254: v93.8,43.07 94.03,43.07 JP1.P$23
  Top 0.3: U2.8 16.71,30.56 16.71,32.08 17.12,32.48 v17.12,41.22
  Bottom 0.3: v93.8,43.07 92.03,41.3 17.2,41.3 v17.12,41.22
IO16_G6  (via drill 0.35)
  Top 0.254: JP1.P$22 93.53,44.05 v93.29,44.05
  Top 0.3: U2.9 17.96,32.04 18.12,32.21 18.12,42.15 v18.08,42.2
  Bottom 0.3: v18.08,42.2 18.22,42.34 91.67,42.34 93.29,43.96 v93.29,44.05
IO17_I2S_SDIN
  Top 0.254: U2.10 19.23,27.79 R4.2
IO18_I2S_LRCLK  (1 unrouted)
  Top 0.254: U2.11 20.74,30.29 20.74,27.96 21.46,27.24
IO19_I2C_SDA  (via drill 0.35)  (1 unrouted)
  Top 0.254: 37.39,28.92 v37.36,28.89 23.56,28.89 23.04,29.41 U2.13 23.04,46.43 v22.63,46.84 | R1.1 42.83,36.73 J6.5 42.83,30.02 v42.66,29.85 | v24.13,67.77 24.13,70.41 24.64,70.92 | J8.2 24.36,71.93 26.61,74.18 106.92,74.18 109.65,71.45 109.65,68.86 109.64,68.87 J4.7
  Bottom 0.254: v37.36,28.89 37.48,29.01 41.82,29.01 v42.66,29.85 | v22.63,46.84 22.63,46.91 18.9,50.65 18.9,64.59 22.07,67.77 v24.13,67.77
IO20_I2C_SCL  (via drill 0.35)
  Top 0.254: J6.3 41.83,36.8 R7.1 40.56,36.98 34.11,30.53 U2.14 23.88,30.96 v23.88,46.79 | v22.02,66.17 22.35,66.5 J8.1 22.36,72.68 24.47,74.79 110,74.79 112.18,72.61 J4.8
  Bottom 0.254: v23.88,46.79 19.99,50.67 19.99,64.15 22.01,66.17 v22.02,66.17
IO21_R6  (via drill 0.35)  (1 unrouted)
  Top 0.3: U2.23 27.32,42.7 v32,47.38 | 97.52,47.92 97.52,44.21 v97.76,43.97
  Bottom 0.3: v97.76,43.97 94.11,47.62 32.16,47.62 32,47.46 v32,47.38
IO38_D  (via drill 0.35)  (1 unrouted)
  Top 0.254: J2.1 46.9,70.35 44.35,70.35 v43.51,71.19 36.77,71.19 19.23,53.64 U2.31 | 102.07,70.79 99.13,73.72 54.55,73.72 v53.65,72.82
  Bottom 0.254: v43.51,71.19 45.39,73.07 53.4,73.07 v53.65,72.82
IO39_HSYNC  (via drill 0.35)
  Top 0.254: JP1.P$9 87.03,45.02 v87,44.99 | U2.32 17.96,47.12 v19.98,45.09
  Bottom 0.254: v87,44.99 86.91,45.07 20,45.07 v19.98,45.09
IO40_DE  (via drill 0.35)
  Top 0.254: JP1.P$7 86.03,47.8 86.03,46.1 v85.73,45.8 | U2.33 16.69,47 v17.73,45.95
  Bottom 0.254: v17.73,45.95 17.82,45.87 85.66,45.87 v85.73,45.8
IO41_VSYNC  (via drill 0.35)
  Top 0.254: v85.51,44.28 85.51,44.54 86.53,45.56 JP1.P$8 | U2.34 15.42,47.16 18.13,44.45 v19.05,44.45
  Bottom 0.254: v85.51,44.28 v85.5,44.28 19.22,44.28 v19.05,44.45
IO42-I2S_BCLK  (via drill 0.35)
  Top 0.254: U2.35 14.15,47.45 17.97,43.62 20.24,43.62 20.91,42.95 v20.91,38.58 | v19.98,28.84 19.99,28.83 19.99,27.3 R19.2
  Bottom 0.254: v20.91,38.58 20.99,38.5 20.99,29.85 v19.98,28.84
IO45_R3  (via drill 0.35)  (1 unrouted)
  Top 0.254: v29.76,48.99 29.79,48.97 31.04,48.97 R31.2
  Top 0.3: U2.26 27.3,46.53 v29.76,48.99 | v98.92,49.6 99.04,49.49 99.04,47.94
  Bottom 0.3: v98.92,49.6 98.59,49.94 30.71,49.94 v29.76,48.99
IO46_B5  (via drill 0.35)  (1 unrouted)
  Top 0.3: U2.16 26.63,33.81 30.33,37.52 v30.33,37.68 | v89.75,37.75 89.75,37.83 90.02,38.11 90.02,48.17
  Bottom 0.3: v30.33,37.68 30.51,37.86 89.64,37.86 v89.75,37.75
IO47_R5  (via drill 0.35)  (1 unrouted)
  Top 0.3: v30.69,47.41 27.25,43.97 U2.24 | 98.03,47.95 98.03,45.09 v98.33,44.79
  Bottom 0.3: v98.33,44.79 94.86,48.26 31.53,48.26 v30.69,47.41
IO48_R4  (via drill 0.35)  (1 unrouted)
  Top 0.3: U2.25 26.06,45.49 27.31,45.49 v29.72,47.9 | 98.54,48.05 98.54,46.08 v98.83,45.79
  Bottom 0.3: v98.83,45.79 95.58,49.03 30.85,49.03 v29.72,47.9
LCD_LEDA  (1 unrouted)
  Top 0.3: JP1.P$39 102.03,53.2 102.03,54.06 | 102.48,53.17 102.11,53.55
  Top 0.5: 102.03,54.06 100.53,55.56 100.53,56.71 101.6,57.79 C21.2 102.76,59.44 C19.2 100.82,59.63 99.57,58.37 98.43,58.37 97.77,59.04 97.77,59.72 U4.5 | D6.2 102.02,53.38
  Top 1: D6.2 102.2,53.2 102.03,53.2
  pour Top: 101.13,51.94 103.31,51.94 102.39,51.02 102.39,49.59 102.18,49.38 101.55,50.01 101.55,51.18 101.13,51.6
LCD_LEDK  (via drill 0.35)
  Top 0.3: 102.53,48.31 104.87,50.65
  Top 0.5: v99.62,57.1 99.57,57.15 U4.3 | R29.1 101.54,56.36 v101.53,56.35
  Bottom 0.5: v101.53,56.35 100.77,57.1 v99.62,57.1
  pour Top: 102.39,56.9 103.14,56.9 103.48,56.56 103.48,55.97 105.08,54.38 105.08,49.36 102.87,47.15 102.56,47.15 102.39,47.32 102.39,48.66 103.82,50.09 103.82,54.8 102.81,55.8 102.39,55.8 102.22,55.97 102.22,56.73
LRCLK
  Top 0.3: U11.2 21.35,23.15 21.35,25.54 R12.1
N$1
  Top 0.3: R3.1 132.03,30.28 LED1.+
N$2
  Top 0.5: U11.5 18.89,14.82 C27.2
N$3
  Top 0.5: C14.1 22.94,13.22 C28.1 21.83,12.12 J5.P$2
N$7
  Top 0.3: JP1.P$10 87.53,52.53 R25.2
N$8
  Top 0.5: U11.8 22.7,14.96 C28.2
N$11
  Top 0.3: J3.A5 125.93,38.35 R13.2
N$13  (1 unrouted)
  Top 0.8: U1.3 111.4,44.81
N$15
  Top 0.5: C16.1 17.39,13.21 C27.1 19.83,12.18 J5.P$1
N$16  (1 unrouted)
  Top 0.8: L5.2 92.06,57.15 U4.1 96.79,52.67 96.8,52.66
N$17
  Top 0.3: J3.B5 125.73,41.34 R14.1
N$20
  Top 0.5: R21.1 116.94,48.44 117.01,48.36 R20.2 116.92,48.38 116.92,47.8 U1.5
N$21  (via drill 0.5)
  Top 0.5: v118.47,23.22 119.29,24.04 R44.2
  Top 0.8: Q3.1 116.14,25.51 v116.23,25.6 | R44.2 R2.1
  Bottom 0.8: v118.47,23.22 118.47,23.37 v116.23,25.6
N$22
  Top 0.8: U26.5 112.76,35.03 R6.1
N$23  (1 unrouted)
  Top 0.8: Q5.1 98.69,62.27 R11.1
N$27
  Top 0.8: Q6.3 81.24,63.4 R48.2 81.56,63.09 Q4.1
N$32
  Top 0.5: R75.1 126.05,50.04 126.05,51.1 Q9.1
N$33
  Top 0.8: R55.2 R54.1 83.09,57.84 Q6.1
N$36
  Top 0.8: Q30.1 89.19,62.66 R172.2 92.44,62.66 Q5.3
N$38
  Top 0.5: R74.1 122.77,49.36 Q10.1
N$40
  Top 0.3: R72.2 115.29,65.55 118.48,65.55 U6.2
N$42
  Top 0.3: U6.3 115.27,64.2 R71.2
N$47
  Top 0.3: SD1.1 117.83,15.46 117.83,15.69 119.12,16.97 R16.2
N$48
  Top 0.3: SD1.8 110.16,17.07 108.89,18.35 R17.2
RTS  (via drill 0.5)
  Top 0.5: R74.2 127.59,49.25 v127.59,50.76 127.57,50.79 127.95,51.17 Q9.2 | v125.99,63.95 125.74,64.2 U6.14
  Bottom 0.5: v127.59,50.76 125.91,52.44 125.91,63.87 v125.99,63.95
TFT-3V3
  Top 0.3: C3.1 93.6,54.13 93.88,54.13 94.54,53.47 94.54,51.93 95.74,50.72 99.61,50.72 101.03,49.31 JP1.P$37
  Top 0.8: Q4.3 81.49,58.72 R56.2 81.49,56.91 82.58,55.83 87.02,55.83 87.6,55.25 R25.1 C23.2 C15.2 C10.2 93.6,54.13
TP_RST
  Top 0.254: J6.7 43.83,35.71 45.03,36.9 R5.2
UART0_RXD0  (via drill 0.35)
  Top 0.254: U2.36 12.88,51.47 v27.14,65.74 v27.15,65.74 | R72.1 113.52,66.13 113.29,65.9 112.09,65.9 v111.85,66.14
  Top 0.3: J10.1 71.36,70.12 v71.36,67.97
  Bottom 0.254: v27.15,65.74 29.42,68 71.33,68 v71.36,67.97 71.4,68.01 109.98,68.01 v111.85,66.14
UART0_TXD0  (via drill 0.35)
  Top 0.254: v29.87,66.8 26.04,66.8 11.61,52.17 U2.37 | v111.73,64.52 111.75,64.49 113.49,64.49 R71.1 | v73.36,66.79 73.36,70.12 J10.2
  Bottom 0.254: v29.87,66.8 29.93,66.86 73.28,66.86 v73.36,66.79 109.45,66.79 v111.73,64.52
USB_D+
  Top 0.254: R9.2 121.57,42.58 121.57,60.16 120.06,61.66 U6.5
USB_D-  (1 unrouted)
  Top 0.254: R8.2 120.65,41.7 120.65,57.74 120.65,59.45 119.69,60.41 118.67,60.41
VBUS  (via drill 0.35)  (5 unrouted)
  Top 0.3: R2.2 121.65,25.57 121.64,25.58 v122.76,25.58 | 119.63,34.02 121.66,34.02 122.71,32.97 v122.78,32.97
  Top 0.6: 129.37,37.2 127.4,37.2 | 129.09,42 130.01,42 131.37,40.64 131.37,38.56 130.01,37.2 129.09,37.2
  Top 0.8: U26.4 116.3,33.59 C50.1 117.99,33.55 C49.2 119.15,33.53 119.63,34.02 120.32,34.7 120.32,35.69 | 120.32,35.69 120.32,36.79 118.85,38.26 D3.1 | 120.32,35.69 125.88,35.69 127.4,37.2
  Bottom 0.3: v122.78,32.97 122.76,32.94 v122.76,25.58
VDD  (via drill 0.5)
  Top 0.8: R10.2 R45.2 C24.1 27.15,15.22 C25.1 25.65,15.11 v25.61,15.15 | v20.32,15.23 20.16,15.39 U11.6
  Bottom 0.8: v25.61,15.15 20.4,15.15 v20.32,15.23
VIN  (via drill 0.5)  (1 unrouted)
  Top 0.5: U1.1 116.11,46.71 U1.4
  Top 0.8: Q30.2 88.95,64.43 88.99,64.39 90.67,64.39 R172.1 91.13,64.44 v92.07,64.44 | 118.86,44.81 119.44,45.39 119.44,53.13 113.54,59.04 v113.54,59.06 | R45.1 33.54,18.22 39.6,24.28 105.15,24.28 v105.22,24.21 | U1.4 118.01,44.66 116.87,43.51 116.87,43.1 C42.2 116.91,42.99 C6.2 116.38,41.33 D3.2 111,38.26 108.78,36.04 v108.78,27.15 109.38,27.75 D5.C 113.46,27.14 113.46,24.69 114.64,23.51 Q3.2
  Top 1: U1.4 118.86,44.81
  Bottom 0.8: v113.54,59.06 111.11,61.49 94.96,61.49 92.07,64.39 v92.07,64.44 | 105.13,24.14 108.1,24.14 108.78,24.83 v108.78,27.15
VIN2  (1 unrouted)
  Top 0.8: U4.6 91.84,59.75 L5.1 91.63,59.54 C18.2 86.5,59.58 Q30.3

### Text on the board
tPlace: J4 | www.elecrow.com
tNames: GND | 3V3 | NC | IO38 | GND | 3V3 | IO19-SDA | IO20-SCL | IO20-SCL | IO19-SDA | 3V3 | GND | IO38 | NC | 3V3 | GND | IO44-RX0 | IO43-TX0 | 3V3 | GND | GND | 5V | 40 | 1 | V2.0 | 1 | 10 | - | I2S-CTRL | IO18-I2S-LRCLK | IO42-I2S-BCLK | IO17-I2S-SDIN | + | VON- | VOP+
tStop: ESP32 Display-5 Inch | SKU:DIS07050H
